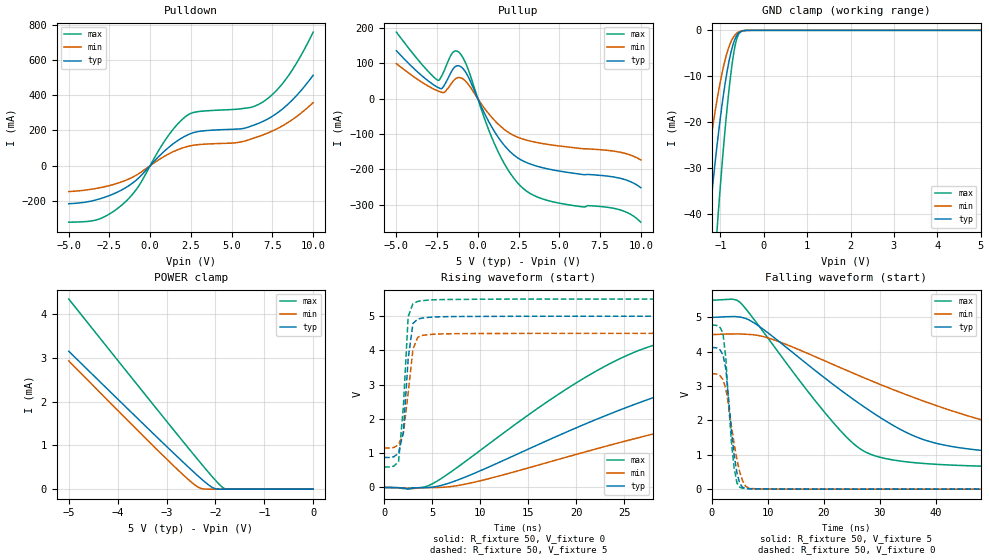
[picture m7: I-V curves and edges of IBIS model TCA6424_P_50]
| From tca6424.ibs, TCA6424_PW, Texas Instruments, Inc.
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[Model]   TCA6424_P_50
Model_type  I/O
Vinl=1.35
Vinh=3.85
Enable   Active-Low
Vref =   0
Rref =   500
Cref =   50p
Vmeas =   2.5
| variable   typ   min   max
C_comp   3.63pF   2.93pF   3.99pF
| C_pullup   6.60pF   2.64pF   9.47pF
| C_pulldown   4.28pF   3.34pF   5.80pF
| C_tri-state   3.63pF   2.93pF   3.99pF
[Temperature Range]   40   100   -40
| Ambient temperature   25   85   -40
[Voltage range]   5   4.5   5.5
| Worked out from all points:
|   slope of the pulldown table from 0 to 0.75 V, typ, clamps not added: 10.5 ohm
|   slope of the pullup table from 0 to 0.75 V, typ, clamps not added: 10.5 ohm
|   GND clamp passes 1 mA (typ) near -0.61 V on its own axis
|   POWER clamp passes 1 mA (typ) near -3.02 V on its own axis
|   rising waveform, R_fixture 50, V_fixture 0: 20-80 % time 23.3ns typ, 32.9ns min, 15.6ns max; typ from 0 V to 4.12 V
|   falling waveform, R_fixture 50, V_fixture 5: 20-80 % time 21.2ns typ, 34.1ns min, 14.2ns max; typ from 5 V to 0.876 V
|   rising waveform, R_fixture 50, V_fixture 5: 20-80 % time 684ps typ, 812ps min, 654ps max; typ from 0.876 V to 5 V
|   falling waveform, R_fixture 50, V_fixture 0: 20-80 % time 1.53ns typ, 2.01ns min, 1.27ns max; typ from 4.12 V to 0 V
[GND Clamp]
| TCA6424_P_50
|   Voltage   I(typ)   I(min)   I(max)
-5V       -590mA     -448.8mA   -795mA
-1.51V    -68.12mA   -45.25mA   -108.4mA
-1.465V   -63.04mA   -41.61mA   -101mA
-1.29V    -44.47mA   -28.47mA   -73.42mA
-1.25V    -40.52mA   -25.71mA   -67.44mA
-1.075V   -24.76mA   -14.94mA   -43.03mA
-1.06V    -23.54mA   -14.13mA   -41.1mA
-920mV    -13.34mA   -7.513mA   -24.47mA
-785mV    -5.952mA   -3.123mA   -11.49mA
-675mV    -2.175mA   -1.137mA   -3.955mA
-565mV    -467.5uA   -292.1uA   -632uA
5V        1.249nA    3.317nA    448pA
[POWER Clamp]
| TCA6424_P_50
|   Voltage   I(typ)   I(min)   I(max)
-5V       3.15mA     2.929mA    4.342mA
-3.24V    1.236mA    953.8uA    1.887mA
-2.49V    439.1uA    160uA      853uA
-2.3V     246.6uA    19.63uA    595.5uA
-2.08V    50.88uA    42.61nA    304.7uA
-1.99V    7.721uA    8.799nA    191.1uA
-1.86V    83.5nA     6.219nA    47.44uA
-1.805V   13.29nA    6.011nA    11.09uA
-1.735V   3.452nA    5.79nA     496nA
-84.45fV  1.249nA    2.537nA    657.8pA
[Pulldown]
| TCA6424_P_50
|   Voltage   I(typ)   I(min)   I(max)
-5V       -216.3mA   -147.4mA   -321.1mA
-3.17V    -190.5mA   -127.2mA   -304.5mA
-1.635V   -132.3mA   -88.14mA   -215.2mA
-695mV    -68.89mA   -45.25mA   -114.4mA
1.14V     103.7mA    66.3mA     173.6mA
2.33V     175.5mA    109.3mA    288.5mA
3.04V     194.5mA    119.6mA    307.4mA
5.175V    206.5mA    128.6mA    318.7mA
6.135V    222mA      148.8mA    329.3mA
7.2V      263.7mA    184.3mA    379.8mA
8.55V     356.6mA    250.3mA    519.1mA
10V       512.8mA    357.4mA    757.3mA
[Pullup]
| TCA6424_P_50
|   Voltage   I(typ)   I(min)   I(max)
-5V       135.9mA    99.31mA    188.6mA
-2.44V    31.7mA     21.81mA    52.05mA
-2.175V   30.45mA    17.66mA    68.46mA
-1.555V   81.88mA    47.36mA    129.8mA
-1.07V    91.37mA    59.47mA    127mA
-620mV    64.88mA    42.88mA    86.27mA
1.22V     -107.1mA   -70.5mA    -147.6mA
2.055V    -153mA     -100.3mA   -215.4mA
2.91V     -179.1mA   -116.2mA   -258.8mA
4.9V      -204mA     -133.2mA   -294.7mA
8.665V    -224.3mA   -150.7mA   -313.6mA
10V       -251.7mA   -173.2mA   -349.4mA
[Ramp]
| TCA6424_P_50
| variable   typ   min   max
dV/dt_r   2.50/2.35E-08   2.04/3.31E-08   2.90/1.57E-08
dV/dt_f   2.49/2.13E-08   2.02/3.41E-08   2.96/1.43E-08
R_load = 50
[Rising Waveform]
| TCA6424_P_50
R_fixture =   50
C_fixture =   0
L_fixture =   0
V_fixture =   0
V_fixture_min = 0
V_fixture_max = 0
|   Time   V(typ)   V(min)   V(max)
0s        3.746nV    27.75nV    804.2pV
5ns       9.165mV    -3.401mV   104.3mV
9.5ns     426.5mV    162mV      976.1mV
19ns      1.62V      887.4mV    2.876V
27ns      2.52V      1.49V      4.051V
33.5ns    3.109V     1.919V     4.439V
44.5ns    3.691V     2.497V     4.631V
67ns      3.99V      3.081V     4.732V
111ns     4.096V     3.3V       4.766V
520ns     4.118V     3.355V     4.771V
[Falling Waveform]
| TCA6424_P_50
R_fixture =   50
C_fixture =   0
L_fixture =   0
V_fixture =   5
V_fixture_min = 4.5
V_fixture_max = 5.5
|   Time   V(typ)   V(min)   V(max)
0s        5V         4.5V       5.5V
5ns       5.008V     4.516V     5.442V
11ns      4.426V     4.351V     4.182V
20.5ns    3.193V     3.71V      2.167V
26ns      2.53V      3.323V     1.231V
31ns      1.99V      2.986V     891.7mV
40.5ns    1.318V     2.409V     719.4mV
63.5ns    985mV      1.537V     628.3mV
105ns     896.1mV    1.237V     602.6mV
520ns     876.2mV    1.153V     598.2mV
[Rising Waveform]
| TCA6424_P_50
R_fixture =   50
C_fixture =   0
L_fixture =   0
V_fixture =   5
V_fixture_min = 4.5
V_fixture_max = 5.5
|   Time   V(typ)   V(min)   V(max)
0s        876.1mV    1.153V     598.2mV
1ns       895.7mV    1.166V     621.7mV
1.5ns     1V         1.25V      752.9mV
2ns       1.614V     1.569V     2.349V
2.5ns     3.752V     2.756V     4.982V
3ns       4.788V     4.04V      5.368V
3.5ns     4.916V     4.384V     5.431V
4ns       4.947V     4.44V      5.455V
5.5ns     4.979V     4.478V     5.481V
520ns     5V         4.5V       5.5V
[Falling Waveform]
| TCA6424_P_50
R_fixture =   50
C_fixture =   0
L_fixture =   0
V_fixture =   0
V_fixture_min = 0
V_fixture_max = 0
|   Time   V(typ)   V(min)   V(max)
0s        4.118V     3.355V     4.771V
1.5ns     4.05V      3.299V     4.702V
2ns       3.909V     3.188V     4.533V
2.5ns     3.511V     2.934V     3.832V
3.5ns     1.715V     1.853V     1.391V
4ns       983.7mV    1.311V     610.2mV
4.5ns     468.5mV    853.7mV    176.7mV
5.5ns     55.18mV    243.8mV    28.68mV
6.5ns     17.66mV    37.94mV    12.63mV
520ns     62.97nV    252nV      35.55nV
